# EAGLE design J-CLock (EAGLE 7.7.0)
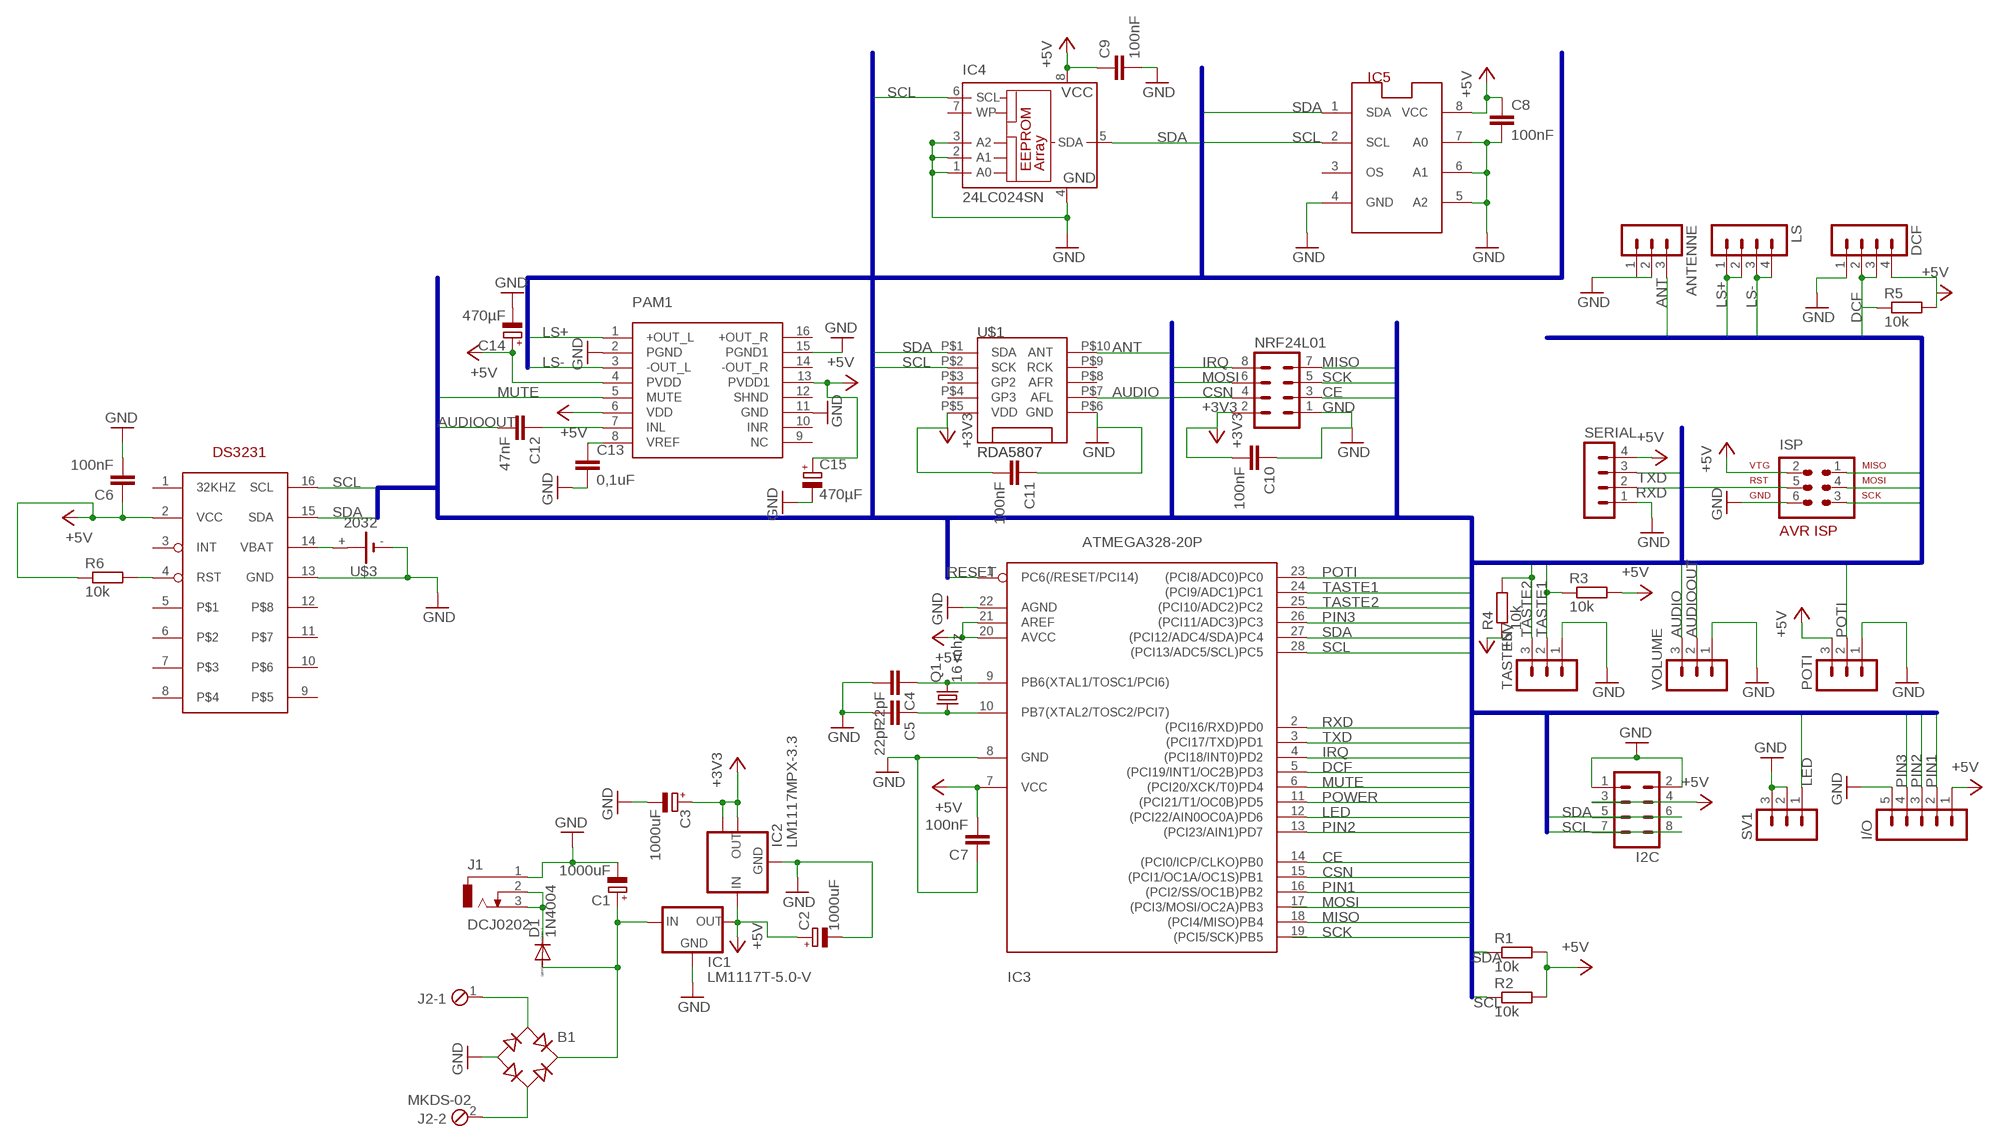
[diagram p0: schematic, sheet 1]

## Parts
ANTENNE  MA03-1  [MA03-1]
B1  B-DIL  [B-DIL]
C1  1000uF  CPOL-EUE5-10.5  [E5-10,5]
C2  1000uF  CPOL-EUE5-10.5  [E5-10,5]
C3  1000uF  CPOL-EUE5-10.5  [E5-10,5]
C4  22pF  C-EU050-030X075  [C050-030X075]
C5  22pF  C-EU050-030X075  [C050-030X075]
C6  100nF  C-EU050-030X075  [C050-030X075]
C7  100nF  C-EU050-030X075  [C050-030X075]
C8  100nF  C-EU050-030X075  [C050-030X075]
C9  100nF  C-EU050-030X075  [C050-030X075]
C10  100nF  C-EU050-030X075  [C050-030X075]
C11  100nF  C-EU050-030X075  [C050-030X075]
C12  47nF  C-EU050-030X075  [C050-030X075]
C13  0,1uF  C-EU050-030X075  [C050-030X075]
C14  470µF  CPOL-EUE3.5-8  [E3,5-8]
C15  470µF  CPOL-EUE3.5-8  [E3,5-8]
D1  1N4004  [DO41-10]
DCF  MA04-1  [MA04-1]
I2C  MA04-2  [MA04-2]
I/O  MA05-1  [MA05-1]
IC1  LM1117T-5.0-V  [TO220V]
IC2  LM1117MPX-3.3  [SOT223]
IC3  ATMEGA328-20P  [DIL28-3]
IC4  24LC024SN  [SO-08]
IC5  LM75_ICN  [SO8_LM75]
ISP  AVR-ISP-6  [AVR-ISP-6]
J1  DCJ0202  [DCJ0202]
J2  MKDS-02  [MKDS-02]
LS  MA04-1  [MA04-1]
NRF24L01  MA04-2  [MA04-2]
PAM1  PAM8403  [SOP-16]
POTI  MA03-1  [MA03-1]
Q1  16 mhz  CRYSTALHC49S  [HC49/S]
R1  10k  R-EU_0207/5V  [0207/5V]
R2  10k  R-EU_0207/5V  [0207/5V]
R3  10k  R-EU_0207/5V  [0207/5V]
R4  10k  R-EU_0207/5V  [0207/5V]
R5  10k  R-EU_0207/5V  [0207/5V]
R6  10k  R-EU_0207/5V  [0207/5V]
SERIAL  MA04-1  [MA04-1]
SV1  MA03-1  [MA03-1]
TASTEN  MA03-1  [MA03-1]
U$1  RDA5807  [RDA]
U$2  DS3231  [SO16]
U$3  2032  [KZH20SMD]
VOLUME  MA03-1  [MA03-1]

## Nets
+3V3: C3.+ C10.2 C11.2 IC2.2(OUT) IC2.TAB(OUT1) NRF24L01.2 U$1.P$5(VDD)
+5V: C2.+ C6.1 C7.2 C8.1 C9.1 C14.+ C15.+ DCF.4 I2C.3 I2C.4 I/O.1 IC1.2(OUT) IC2.3(IN) IC3.7(VCC) IC3.20(AVCC) IC3.21(AREF) IC4.8(VCC) IC5.8(VCC) ISP.2 PAM1.4(PVDD) PAM1.6(VDD) PAM1.13(PVDD1) POTI.3 R1.2 R2.2 R3.2 R4.1 R5.2 R6.1 SERIAL.4 U$2.2(VCC)
ANT: ANTENNE.3 U$1.P$10(ANT)
AUDIO: U$1.P$7(AFL) VOLUME.3
AUDIOOUT: C12.2 VOLUME.2
CE: IC3.14((PCI0/ICP/CLKO)PB0) NRF24L01.3
CSN: IC3.15((PCI1/OC1A/OC1S)PB1) NRF24L01.4
DCF: DCF.2 DCF.3 IC3.5((PCI19/INT1/OC2B)PD3) R5.1
GND: ANTENNE.1 ANTENNE.2 B1.- C1.- C2.- C3.- C4.2 C5.2 C6.2 C7.1 C8.2 C9.2 C10.1 C11.1 C13.2 C14.- C15.- DCF.1 I2C.1 I2C.2 I/O.5 IC1.1(GND) IC2.1(GND) IC3.8(GND) IC3.22(AGND) IC4.1(A0) IC4.2(A1) IC4.3(A2) IC4.4(GND) IC5.4(GND) IC5.5(A2) IC5.6(A1) IC5.7(A0) ISP.6 J1.1 NRF24L01.1 PAM1.2(PGND) PAM1.11(GND) PAM1.15(PGND1) POTI.1 SERIAL.1 SV1.2 SV1.3 TASTEN.1 U$1.P$6(GND) U$2.13(GND) U$3.- VOLUME.1
IRQ: IC3.4((PCI18/INT0)PD2) NRF24L01.8
LED: IC3.12((PCI22/AIN0OC0A)PD6) SV1.1
LS+: LS.1 LS.2 PAM1.1(+OUT_L)
LS-: LS.3 LS.4 PAM1.3(-OUT_L)
MISO: IC3.18((PCI4/MISO)PB4) ISP.1 NRF24L01.7
MOSI: ISP.4 NRF24L01.6
MUTE: IC3.6((PCI20/XCK/T0)PD4) PAM1.5(MUTE)
N$1: B1.AC2 J2.2
N$2: C4.1 IC3.9(PB6(XTAL1/TOSC1/PCI6)) Q1.2
N$3: B1.+ C1.+ D1.A IC1.3(IN)
N$4: C5.1 IC3.10(PB7(XTAL2/TOSC2/PCI7)) Q1.1
N$5: U$2.14(VBAT) U$3.+
N$6: D1.C J1.2 J1.3
N$7: B1.AC1 J2.1
N$8: R6.2 U$2.4(RST)
N$9: C12.1 PAM1.7(INL)
N$10: C13.1 PAM1.8(VREF)
PIN1: I/O.2 IC3.16((PCI2/SS/OC1B)PB2)
PIN2: I/O.3 IC3.13((PCI23/AIN1)PD7)
PIN3: I/O.4 IC3.26((PCI11/ADC3)PC3)
POTI: IC3.23((PCI8/ADC0)PC0) POTI.2
POWER: IC3.11((PCI21/T1/OC0B)PD5)
RESET: IC3.1(PC6(/RESET/PCI14)) ISP.5
RXD: IC3.2((PCI16/RXD)PD0) SERIAL.2
SCK: ISP.3 NRF24L01.5
SCL: I2C.7 I2C.8 IC3.28((PCI13/ADC5/SCL)PC5) IC4.6(SCL) IC5.2(SCL) R2.1 U$1.P$2(SCK) U$2.16(SCL)
SDA: I2C.5 I2C.6 IC3.27((PCI12/ADC4/SDA)PC4) IC4.5(SDA) IC5.1(SDA) R1.1 U$1.P$1(SDA) U$2.15(SDA)
TASTE1: IC3.24((PCI9/ADC1)PC1) R3.1 TASTEN.2
TASTE2: IC3.25((PCI10/ADC2)PC2) R4.2 TASTEN.3
TXD: IC3.3((PCI17/TXD)PD1) SERIAL.3
Unconnected: IC3.17((PCI3/MOSI/OC2A)PB3) IC3.19((PCI5/SCK)PB5) IC4.7(WP) IC5.3(OS) PAM1.9(NC) PAM1.10(INR) PAM1.12(SHND) PAM1.14(-OUT_R) PAM1.16(+OUT_R) U$1.P$3(GP2) U$1.P$4(GP3) U$1.P$8(AFR) U$1.P$9(RCK) U$2.1(32KHZ) U$2.3(INT) U$2.5 U$2.6 U$2.7 U$2.8 U$2.9 U$2.10 U$2.11 U$2.12

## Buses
CE,CSN,SCK,MOSI,MISO,IRQ,RESET,SDA,SCL,TXD,RXD,TASTE1,TASTE2,POTI,DCF,MUTE,POWER,LED,AUDIO,AUDIOOUT,LS+,LS-,ANT,PIN1,PIN2,PIN3

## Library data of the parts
ANTENNE POTI SV1 TASTEN VOLUME = con-lstb:MA03-1: PIN HEADER; OC_FARNELL: unknown; OC_NEWARK: unknown
B1 = rectifier:B-DIL: RECTIFIER
C1-C3 C14 C15 = resistor:CPOL-EU: POLARIZED CAPACITOR, European symbol
C4-C13 = resistor:C-EU: CAPACITOR, European symbol
D1 = diode:1N4004: DIODE
DCF LS SERIAL = con-lstb:MA04-1: PIN HEADER; OC_FARNELL: unknown; OC_NEWARK: unknown
I2C NRF24L01 = con-lstb:MA04-2: PIN HEADER; OC_FARNELL: unknown; OC_NEWARK: unknown
I/O = con-lstb:MA05-1: PIN HEADER; OC_FARNELL: unknown; OC_NEWARK: unknown
IC1 = lm1117:LM1117T-*
IC2 = lm1117:LM1117MPX-*
IC3 = atmega328:ATMEGA328*P: MICROCONTROLLER 32 kBytes FLASH 2 kBytes SRAM 1 kBytes EEPROM USART 8-channel 10 bit ADC
IC4 = microchip:24*: Serial EEPROM I2C; MF: MICROCHIP; MPN: 24LC024/SN; OC_FARNELL: 1659744; OC_NEWARK: 92C7092
IC5 = lm75:LM75_IC: Temperatursensor
ISP = avr-6:AVR-ISP-6: AVR ISP-6 Serial Programming Header
J1 = con-jack:DCJ0202: DC POWER JACK Source: DCJ0202.pdf; OC_FARNELL: unknown; OC_NEWARK: unknown
J2 = con-phoenix-500:MKDS-02: MKDSN COMBICON SERIES
PAM1 = PAM8403:PAM8403: Dual channel audio amplifier IC - PAM8403
Q1 = crystal:CRYSTAL: CRYSTAL; OC_FARNELL: 1667008; OC_NEWARK: unknown
R1-R6 = resistor:R-EU_: RESISTOR, European symbol
U$1 = RDA5807:RDA5807
U$2 = DS3231:DS3231
U$3 = kzh20_lithium_batterie_holder:2032

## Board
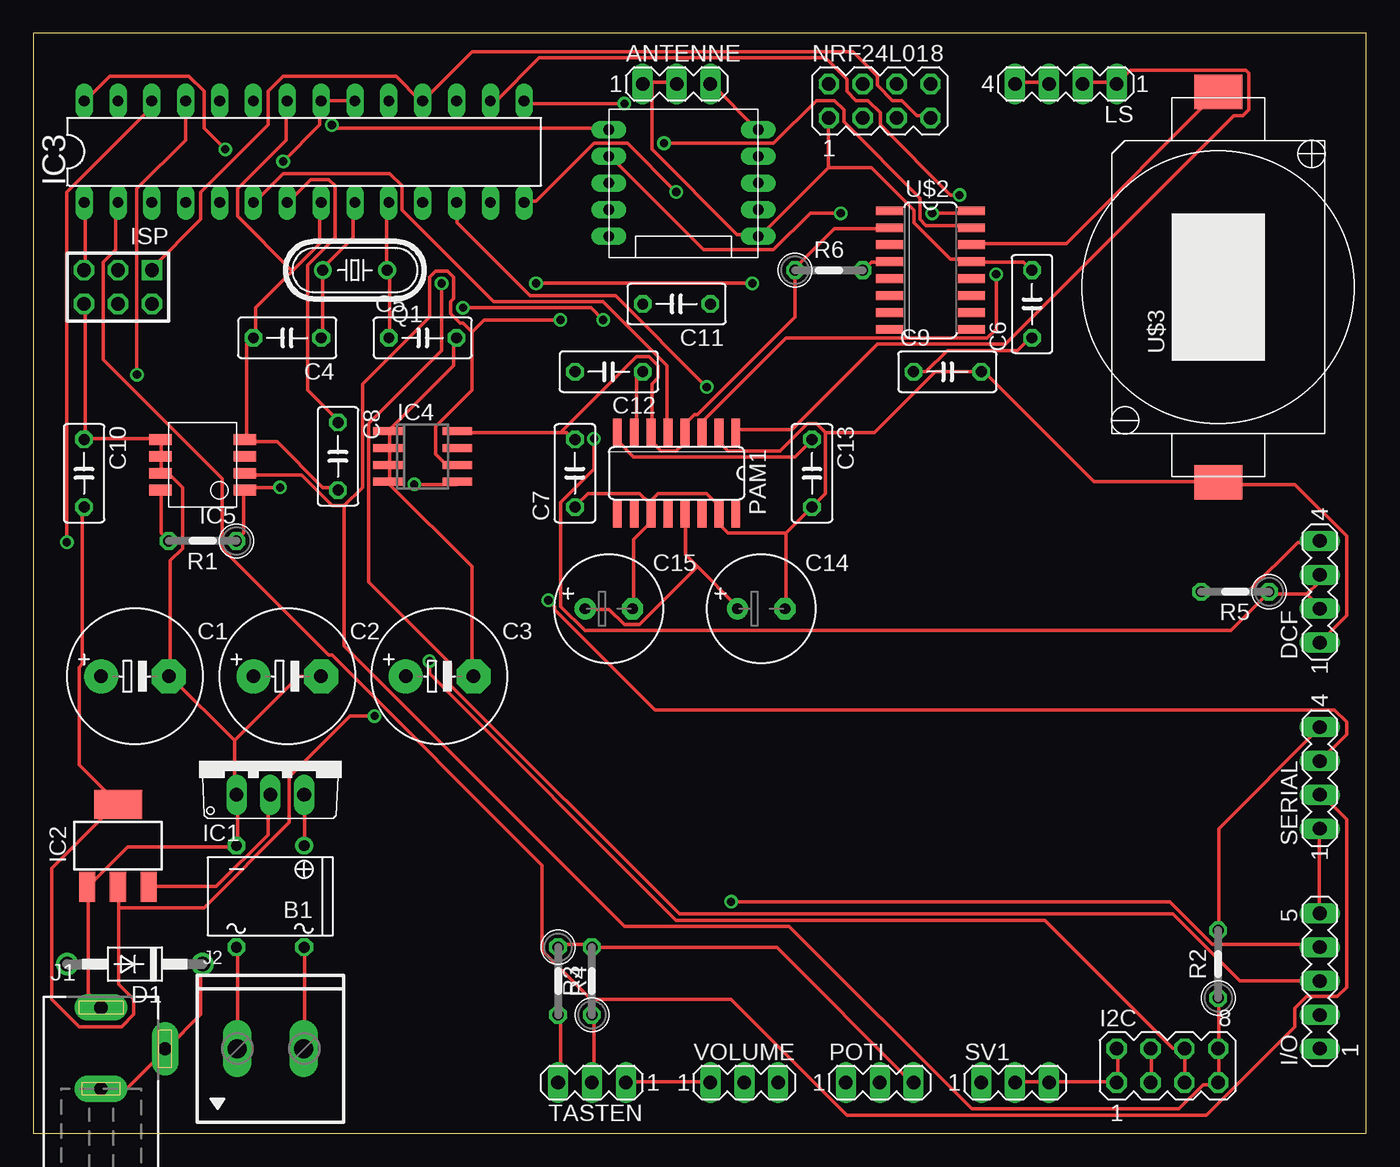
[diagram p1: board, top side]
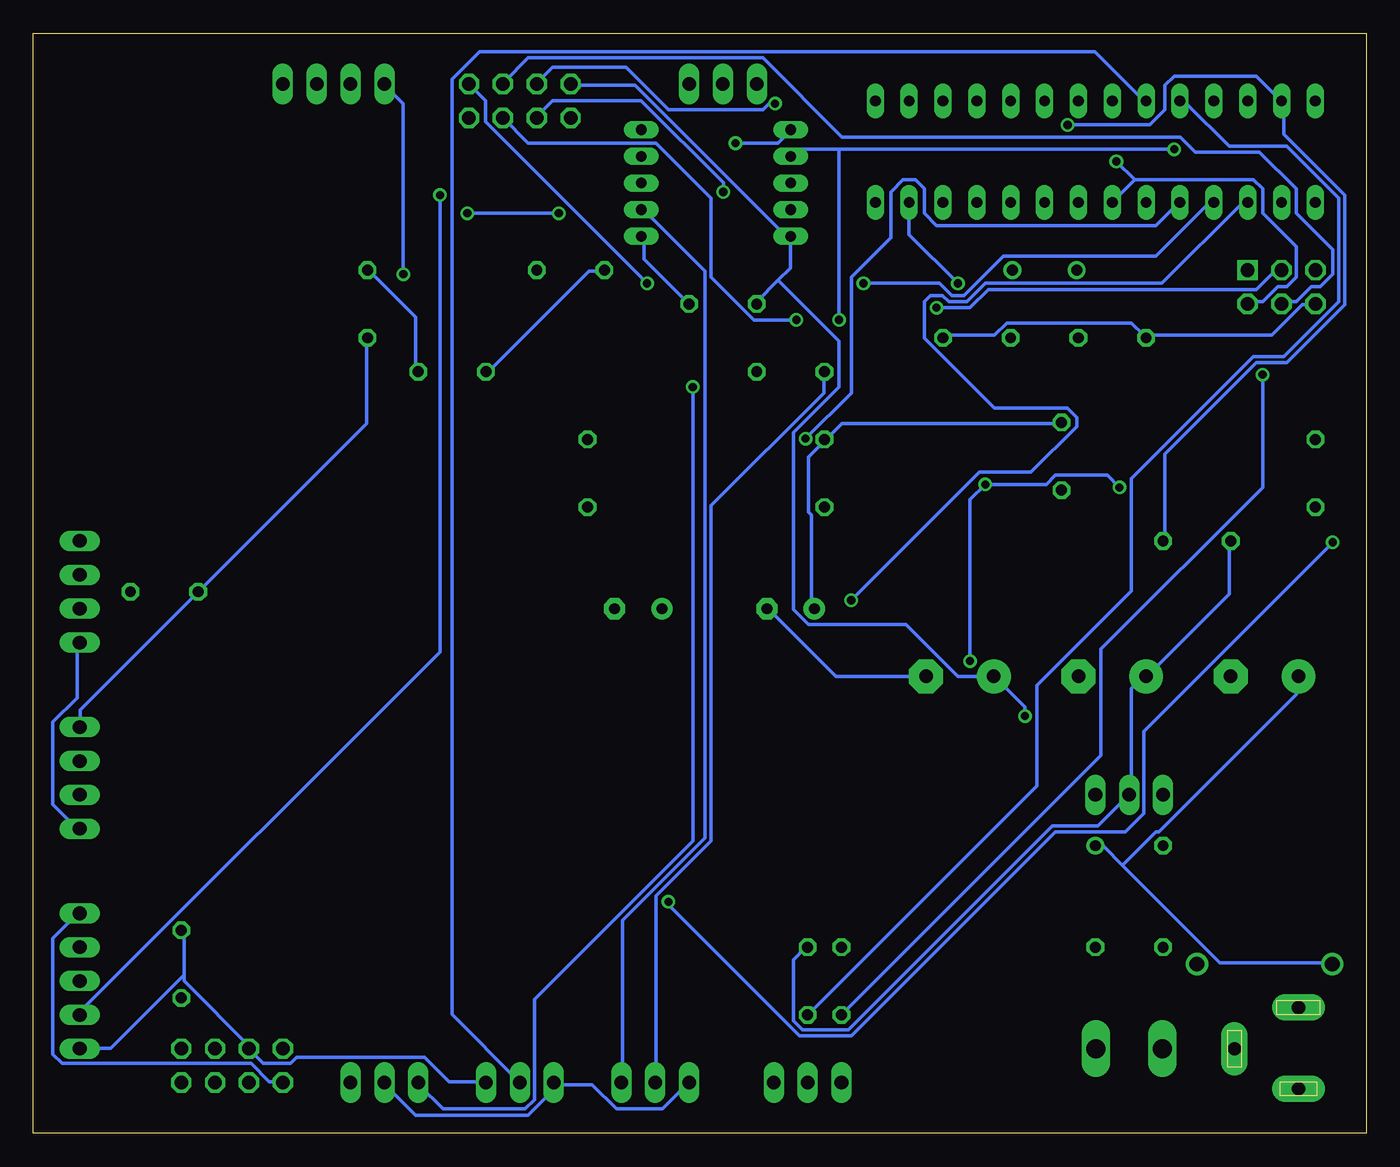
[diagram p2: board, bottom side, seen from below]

Size 100 x 82.54 mm. Coordinates in mm from the lower left corner, seen from the top.
Outline: 0,0 100,0 100,82.54 0,82.54 0,0
Copper layers (1*16): Top 0.035mm / dielectric 1.5mm / Bottom 0.035mm
Design rules "default": minimum track width 10mil, minimum drill 24mil, track to track 8mil, track to pad 8mil, pad to pad 8mil, via to via 8mil, smd to smd 8mil, copper to edge 40mil, drill to drill 8mil, minimum pad ring 10mil, minimum via ring 8mil, stop-mask expansion 4mil, vias tented up to drill 0mil, thermal gap 10mil

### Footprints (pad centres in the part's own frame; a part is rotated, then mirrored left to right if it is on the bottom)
MA03-1 = drill 1.016 long: 1 -2.54,0; 2 0,0; 3 2.54,0
B-DIL = drill 0.813: + -2.54,-3.81 | drill 0.813 octagon: - 2.54,-3.81; AC1 2.54,3.81; AC2 -2.54,3.81
E5-10,5 = drill 1.016 pad 2.54: + -2.54,0 | drill 1.016 pad 2.54 octagon: - 2.54,0
C050-030X075 = drill 0.813 octagon: 1 -2.54,0; 2 2.54,0
E3,5-8 = drill 0.813 pad 1.6: + -1.778,0 | drill 0.813 pad 1.6 octagon: - 1.778,0
DO41-10 = drill 1.118: A 5.08,0; C -5.08,0
MA04-1 = drill 1.016 long: 1 -3.81,0; 2 -1.27,0; 3 1.27,0; 4 3.81,0
MA04-2 = drill 1.016 octagon: 1 -3.81,-1.27; 2 -3.81,1.27; 3 -1.27,-1.27; 4 -1.27,1.27; 5 1.27,-1.27; 6 1.27,1.27; 7 3.81,-1.27; 8 3.81,1.27
MA05-1 = drill 1.016 long: 1 -5.08,0; 2 -2.54,0; 3 0,0; 4 2.54,0; 5 5.08,0
TO220V = drill 1.016 long: 1 -2.54,-2.54; 2 0,-2.54; 3 2.54,-2.54
SOT223 = smd 1.219 x 2.235: 1 -2.311,-3.099; 2 0,-3.099; 3 2.311,-3.099 | smd 3.6 x 2.2: TAB 0,3.099
DIL28-3 = drill 0.813 long: 1 -16.51,-3.81; 2 -13.97,-3.81; 3 -11.43,-3.81; 4 -8.89,-3.81; 5 -6.35,-3.81; 6 -3.81,-3.81; 7 -1.27,-3.81; 8 1.27,-3.81; 9 3.81,-3.81; 10 6.35,-3.81; 11 8.89,-3.81; 12 11.43,-3.81; 13 13.97,-3.81; 14 16.51,-3.81; 15 16.51,3.81; 16 13.97,3.81; 17 11.43,3.81; 18 8.89,3.81; 19 6.35,3.81; 20 3.81,3.81; 21 1.27,3.81; 22 -1.27,3.81; 23 -3.81,3.81; 24 -6.35,3.81; 25 -8.89,3.81; 26 -11.43,3.81; 27 -13.97,3.81; 28 -16.51,3.81
SO-08 = smd 0.6 x 2.2: 1 -1.905,-2.6; 2 -0.635,-2.6; 3 0.635,-2.6; 4 1.905,-2.6; 5 1.905,2.6; 6 0.635,2.6; 7 -0.635,2.6; 8 -1.905,2.6
SO8_LM75 = smd 0.813 x 1.676: 1 -1.27,-3.175; 2 0,-3.175; 3 1.27,-3.175; 4 2.54,-3.175; 5 2.54,3.175; 6 1.27,3.175; 7 0,3.175; 8 -1.27,3.175
AVR-ISP-6 = drill 1.016 square: 1 -2.54,-1.27 | drill 1.016 octagon: 2 -2.54,1.27; 3 0,-1.27; 4 0,1.27; 5 2.54,-1.27; 6 2.54,1.27
DCJ0202 = drill 1 pad 2 long: 1 0,3.1; 2 4.8,0; 3 0,-3
MKDS-02 = drill 1.422 long: 1 -2.5,0; 2 2.5,0
SOP-16 = smd 0.66 x 2.032: 1 -4.445,-3.073; 2 -3.175,-3.073; 3 -1.905,-3.073; 4 -0.635,-3.073; 5 0.635,-3.073; 6 1.905,-3.073; 7 3.175,-3.073; 8 4.445,-3.073; 9 4.445,3.073; 10 3.175,3.073; 11 1.905,3.073; 12 0.635,3.073; 13 -0.635,3.073; 14 -1.905,3.073; 15 -3.175,3.073; 16 -4.445,3.073
HC49/S = drill 0.813: 1 -2.413,0; 2 2.413,0
0207/5V = drill 0.813 octagon: 1 -2.54,0; 2 2.54,0
RDA = drill 0.8 pad 1.265 long: P$1 0,8; P$2 0,6; P$3 0,4; P$4 0,2; P$5 0,0; P$6 11.2,0; P$7 11.2,2; P$8 11.2,4; P$9 11.2,6; P$10 11.2,8
SO16 = smd 0.66 x 2.032: 1 -4.445,-3.073; 2 -3.175,-3.073; 3 -1.905,-3.073; 4 -0.635,-3.073; 5 0.635,-3.073; 6 1.905,-3.073; 7 3.175,-3.073; 8 4.445,-3.073; 9 4.445,3.073; 10 3.175,3.073; 11 1.905,3.073; 12 0.635,3.073; 13 -0.635,3.073; 14 -1.905,3.073; 15 -3.175,3.073; 16 -4.445,3.073
KZH20SMD = smd 2.6 x 3.6: + 14.65,0; - -14.65,0

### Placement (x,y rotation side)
ANTENNE  48.26,78.74 0 top
B1  17.78,17.78 180 top
C1  7.62,34.29 0 top
C2  19.05,34.29 0 top
C3  30.48,34.29 0 top
C4  19.05,59.69 180 top
C5  29.21,59.69 0 top
C6  74.93,62.23 90 top
C7  40.64,49.53 90 top
C8  22.86,50.8 270 top
C9  68.58,57.15 0 top
C10  3.81,49.53 270 top
C11  48.26,62.23 180 top
C12  43.18,57.15 180 top
C13  58.42,49.53 270 top
C14  54.61,39.37 0 top
C15  43.18,39.37 0 top
D1  7.62,12.7 180 top
DCF  96.52,40.64 90 top
I2C  85.09,5.08 0 top
I/O  96.52,11.43 90 top
IC1  17.78,27.94 0 top
IC2  6.35,21.59 0 top
IC3  20.32,73.66 0 top
IC4  29.21,50.8 270 top
IC5  12.7,49.53 90 top
ISP  6.35,63.5 180 top
J1  5.08,6.35 0 top
J2  17.78,6.35 0 top
LS  77.47,78.74 180 top
NRF24L01  63.5,77.47 0 top
PAM1  48.26,49.53 180 top
POTI  63.5,3.81 0 top
Q1  24.13,64.77 180 top
R1  12.7,44.45 180 top
R2  88.9,12.7 90 top
R3  41.91,11.43 90 top
R4  39.37,11.43 270 top
R5  90.17,40.64 180 top
R6  59.69,64.77 0 top
SERIAL  96.52,26.67 90 top
SV1  73.66,3.81 0 top
TASTEN  41.91,3.81 180 top
U$1  43.18,67.31 0 top
U$2  67.31,64.77 270 top
U$3  88.9,63.5 90 top
VOLUME  53.34,3.81 0 top

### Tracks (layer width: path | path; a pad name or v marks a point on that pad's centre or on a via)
+3V3  (via drill 0.61)
  Top 0.254: 6.4,16.92 6.4,11.2 7.54,10.06 7.54,8.91 6.63,8 3.43,8 1.37,10.06 1.37,19.89 6.17,24.69 IC2.TAB 6.17,24.92 3.43,27.66 3.43,34.98 3.66,35.2 3.66,46.86 C10.2 | 6.4,16.92 6.4,18.29 IC2.2 | 6.4,16.92 12.8,16.92 19.2,23.32 19.2,26.75 23.77,31.32 v25.6,31.32
  Bottom 0.254: 43.2,66.98 43.2,64.92 44.12,64.01 | 43.2,66.98 43.2,67.21 U$1.P$5 43.2,66.98 | 44.12,64.01 45.72,62.41 C11.2 | 43.2,66.98 54.86,78.64 59.66,78.64 NRF24L01.2 | 44.12,64.01 39.55,59.44 39.55,56.01 42.98,52.58 42.98,39.32 41.83,38.18 34.52,38.18 30.63,34.29 C3.+ 27.89,34.29 25.6,32 v25.6,31.32
+5V  (via drill 0.61)
  Top 0.254: U$2.2 64.24,67.89 60.12,67.89 57.15,64.92 R6.1 57.15,61.27 49.84,53.95 49.61,53.95 48.92,53.26 48.92,52.81 PAM1.4 48.69,52.58 48.69,51.66 48.23,51.21 47.09,51.21 46.41,51.89 46.41,52.58 PAM1.6 46.41,52.81 46.41,56.24 46.86,56.69 46.86,57.61 46.18,58.29 45.26,58.29 39.55,52.58 | C9.1 66.98,57.15 68.58,58.75 73.84,58.75 74.75,59.66 C6.1 | 49.84,42.52 52.81,39.55 C14.+ | 49.84,42.52 48.92,43.43 48.92,46.41 PAM1.13 | 49.84,42.52 45.49,38.18 44.35,38.18 43.2,39.32 41.6,39.32 C15.+ | IC3.20 24,77.5 21.72,77.5 IC3.21 21.49,77.27 21.49,75.67 v18.75,72.92 | 39.55,52.58 40.01,52.58 40.46,52.12 C7.2 | 39.55,52.58 32,52.58 IC4.8 | IC3.7 19.2,69.95 20.8,71.55 22.17,71.55 22.63,71.09 22.63,67.21 20.57,65.15 20.57,55.78 22.86,53.49 C8.1 | IC2.3 8.69,18.52 13.72,18.52 17.6,22.4 17.6,25.38 IC1.2 | IC5.8 9.6,48.23 9.6,45.03 10.06,44.58 R1.2 | R5.2 87.78,40.69 91.21,40.69 94.87,44.35 96.47,44.35 DCF.4 | R4.1 39.55,14.17 41.83,14.17 R3.2 42.06,13.95 55.78,13.95 65.84,3.89 POTI.3 | I2C.3 83.9,3.89 83.9,6.17 I2C.4 | SERIAL.4 96.47,30.4 88.92,22.86 88.92,15.32 R2.2
  Bottom 0.254: R6.1 57.15,64.69 58.29,64.69 65.84,57.15 C9.1 | C8.1 22.86,53.26 39.32,53.26 40.46,52.12 C7.2 40.69,51.89 41.83,50.75 41.83,46.63 41.6,46.41 41.6,39.55 C15.+ | 17.37,71.55 8.46,71.55 7.77,70.87 7.77,69.04 5.26,66.52 5.26,64.24 5.94,63.55 6.63,63.55 7.77,62.41 8.69,62.41 ISP.2 | 17.37,71.55 18.97,69.95 IC3.7 | 17.37,71.55 v18.75,72.92 | R1.2 10.29,44.35 10.29,40.46 16.46,34.29 C2.+ 16.69,34.29 17.6,33.38 17.6,25.6 IC1.2 17.83,25.38 20.12,23.09 23.55,23.09 38.86,7.77 42.29,7.77 42.98,8.46 42.98,13.03 42.06,13.95 R3.2 | SERIAL.4 96.47,30.63 96.47,31.77 87.78,40.46 R5.2 87.55,40.69 74.98,53.26 74.98,59.66 C6.1 | 88.7,11.89 88.7,11.43 83.67,6.4 I2C.4 83.67,6.17 82.75,5.26 80.7,5.26 80.24,5.71 70.64,5.71 68.81,3.89 66.06,3.89 POTI.3 | 88.7,11.89 88.7,15.09 R2.2 | 88.7,11.89 94.18,6.4 96.47,6.4 I/O.1
ANT
  Top 0.254: U$1.P$10 54.18,75.44 50.98,78.64 ANTENNE.3
AUDIO
  Bottom 0.254: U$1.P$7 54.18,69.27 49.61,64.69 49.61,22.17 55.78,16 55.78,3.89 VOLUME.3
AUDIOOUT
  Bottom 0.254: C12.2 40.69,57.15 40.69,55.55 49.15,47.09 49.15,21.95 53.26,17.83 53.26,3.89 VOLUME.2
CE  (via drill 0.61)
  Top 0.254: v48.23,70.64 44.58,74.3 42.06,74.3 37.72,69.95 37.03,69.95 IC3.14
  Bottom 0.254: v48.23,70.64 48.23,71.32 54.41,77.5 61.04,77.5 62.18,76.35 NRF24L01.3
CSN  (via drill 0.61)
  Top 0.254: v44.35,77.27 37.03,77.27 IC3.15
  Bottom 0.254: v44.35,77.27 44.81,77.27 45.26,76.81 52.35,76.81 55.55,80.01 61.04,80.01 62.18,78.87 NRF24L01.4
DCF  (via drill 0.61)
  Top 0.254: 95.56,40.46 92.81,40.46 R5.1 92.58,40.46 89.84,37.72 41.38,37.72 39.55,39.55 39.55,47.32 42.06,49.84 v42.06,52.12 | 95.56,40.46 96.47,39.55 DCF.2 | 95.56,40.46 96.47,41.38 96.47,41.83 DCF.3
  Bottom 0.254: v42.06,52.12 38.63,55.55 38.63,64.24 35.66,67.21 35.66,70.64 34.75,71.55 33.83,71.55 33.15,70.87 33.15,69.04 32.23,68.12 15.77,68.12 14.17,69.72 IC3.5
GND
  Top 0.254: SV1.2 73.84,3.89 76.12,3.89 SV1.3 76.35,3.89 81.15,3.89 I2C.1 81.38,3.89 81.38,6.17 I2C.2 | TASTEN.1 44.58,3.89 50.75,3.89 VOLUME.1 | I/O.5 96.47,16.69 96.47,22.86 SERIAL.1 | DCF.1 96.7,37.03 98.53,38.86 98.53,44.81 94.64,48.69 88.92,48.69 U$3.- 88.7,48.92 79.55,48.92 71.32,57.15 C9.2 67.67,57.15 63.09,52.58 59.44,52.58 | 46.18,47.32 46.18,46.63 PAM1.11 | 46.18,47.32 45.49,48.01 41.6,48.01 40.69,47.09 C7.1 | 46.18,47.32 46.86,48.01 50.52,48.01 51.44,47.09 PAM1.15 51.44,45.72 52.12,45.03 56.46,45.03 | 46.18,47.32 PAM1.11 | C15.- 45.03,39.55 45.03,44.58 46.18,45.72 46.18,46.41 PAM1.11 | 46.41,78.87 48.23,78.87 ANTENNE.2 | 46.41,78.87 45.72,78.87 ANTENNE.1 46.41,78.87 | 59.66,72.47 59.66,76.12 NRF24L01.1 | 59.66,72.47 54.41,67.21 U$1.P$6 54.18,67.44 52.81,67.44 46.41,73.84 46.41,78.87 | C6.2 74.75,64.92 74.3,65.38 70.41,65.38 U$2.13 70.18,65.61 68.81,65.61 66.06,68.35 66.06,69.27 62.87,72.47 59.66,72.47 | PAM1.2 51.44,51.89 52.12,51.21 56.01,51.21 58.06,53.26 58.75,53.26 59.44,52.58 | 59.44,52.58 59.44,48.01 C13.2 56.46,45.03 | 56.46,45.03 56.46,39.55 C14.- | J1.1 5.03,9.6 4.12,10.52 4.12,18.29 IC2.1 4.12,18.52 7.09,21.49 15.09,21.49 B1.- 15.32,21.72 15.32,25.38 IC1.1 15.09,25.6 15.09,29.49 | 10.29,34.29 15.09,29.49 | C2.- 19.89,34.29 15.09,29.49 | 3.89,52.12 9.37,52.12 IC5.5 9.6,51.89 9.6,50.98 IC5.6 9.6,50.75 9.6,49.61 IC5.7 9.6,49.38 10.29,49.38 11.2,48.46 11.2,43.89 10.29,42.98 10.29,34.29 | 3.89,52.12 3.89,62.18 ISP.6 | 3.89,52.12 C10.1 | 26.75,51.44 26.75,52.58 IC4.1 26.75,52.81 31.55,57.61 31.55,59.66 C5.2 | 26.75,51.44 26.75,50.29 IC4.3 26.75,50.06 26.75,48.92 IC4.4 26.75,48.69 32.92,42.52 32.92,34.29 C3.-
  Top 0.254: 26.75,51.44 IC4.2 | C8.2 22.86,48.46 21.72,48.46 18.29,51.89 16,51.89 IC5.4 16,52.12 16,59.21 16.46,59.66 C4.2 16.69,59.89 16.69,61.95 19.43,64.69 | 19.43,64.69 21.49,66.75 21.49,69.72 IC3.8 | 19.43,64.69 15.32,68.81 15.32,70.87 18.97,74.52 18.97,77.27 IC3.22 | 10.29,34.29 C1.-
  Bottom 0.254: 60.58,3.66 58.06,3.66 56.24,1.83 52.81,1.83 50.98,3.66 VOLUME.1 | 60.58,3.66 60.81,3.66 POTI.1 60.58,3.66 | 60.58,3.66 62.87,1.37 71.32,1.37 73.61,3.66 SV1.2 | DCF.1 96.7,36.8 96.7,32.69 98.53,30.86 98.53,24.69 96.7,22.86 SERIAL.1 | I2C.1 81.38,3.89 82.3,3.89 83.67,5.26 97.84,5.26 98.53,5.94 98.53,14.63 96.7,16.46 I/O.5 | C3.- 39.78,34.29 44.81,39.32 C15.- | C11.1 54.18,65.61 54.18,67.21 U$1.P$6 | C9.2 71.32,57.15 71.32,61.27 74.75,64.69 C6.2 | C5.2 31.55,59.89 27.89,59.89 26.98,60.81 17.6,60.81 16.69,59.89 C4.2 16.46,59.89 7.09,59.89 4.8,62.18 3.89,62.18 ISP.6
IRQ  (via drill 0.61)
  Top 0.254: v53.95,63.78 v37.72,63.78
  Bottom 0.254: v37.72,63.78 32,63.78 31.09,62.87 30.18,62.87 27.2,65.84 15.77,65.84 11.89,69.72 11.43,69.72 IC3.4 | v53.95,63.78 66.06,75.89 66.06,77.5 NRF24L01.8
LED  (via drill 0.61)
  Top 0.254: v50.52,56.01 43.66,62.87 37.26,62.87 31.77,68.35 31.77,69.72 IC3.12
  Bottom 0.254: v50.52,56.01 50.52,21.95 62.41,10.06 62.41,2.52 63.09,1.83 69.27,1.83 71.09,3.66 SV1.1
LS+
  Top 0.254: PAM1.1 52.81,52.81 56.92,52.81 63.32,59.21 72.92,59.21 90.07,76.35 90.75,76.35 91.21,76.81 91.21,79.55 90.98,79.78 82.3,79.78 81.38,78.87 LS.1 81.15,78.87 78.87,78.87 LS.2
LS-  (via drill 0.61)
  Top 0.254: v72.24,64.47 72.24,60.35 71.55,59.66 56.46,59.66 50.29,53.49 50.29,52.81 PAM1.3 | LS.3 76.12,78.87 73.84,78.87 LS.4
  Bottom 0.254: v72.24,64.47 72.24,77.27 73.61,78.64 LS.4
MISO
  Top 0.254: ISP.1 8.91,64.92 12.57,68.58 12.57,70.64 17.6,75.67 17.6,78.18 18.75,79.32 27.2,79.32 29.03,77.5 IC3.18 29.26,77.5 32.92,81.15 61.49,81.15 63.32,79.32 63.32,78.64 64.47,77.5 65.15,77.5 66.29,76.35 67.21,76.35 NRF24L01.7
MOSI
  Bottom 0.254: ISP.4 6.17,62.41 5.26,62.41 4.12,63.55 3.43,63.55 2.52,64.47 2.52,66.29 5.26,69.04 5.26,70.87 8,73.61 12.8,73.61 13.95,74.75 39.32,74.75 45.26,80.7 62.87,80.7 64.69,78.87 NRF24L01.6
MUTE
  Top 0.254: PAM1.5 47.55,52.81 47.55,57.61 42.75,62.41 34.52,62.41 27.66,69.27 27.66,71.09 26.75,72.01 18.75,72.01 16.69,69.95 IC3.6
N$1
  Top 0.254: B1.AC2 20.34,13.95 20.34,6.4 J2.2
N$2
  Top 0.254: C4.1 21.72,59.89 Q1.2 21.72,64.92 24,67.21 24,69.72 IC3.9
N$3
  Top 0.254: B1.+ 20.34,21.72 20.34,25.38 IC1.3
  Bottom 0.254: 18.29,20.12 19.66,21.49 20.12,21.49 B1.+ | 18.29,20.12 10.97,12.8 2.74,12.8 D1.A | 18.29,20.12 15.77,22.63 15.54,22.63 5.26,32.92 5.26,34.29 C1.+
N$4
  Top 0.254: IC3.10 26.52,69.72 26.52,64.92 Q1.1 26.75,64.69 26.75,59.89 C5.1
N$5
  Top 0.254: U$2.14 70.41,66.75 77.5,66.75 88.7,77.95 U$3.+
N$6
  Top 0.254: D1.C 12.57,12.57 12.57,8.91 10.06,6.4 J1.2 9.83,6.17 7.09,3.43 5.26,3.43 J1.3
N$7
  Top 0.254: B1.AC1 15.32,13.95 15.32,6.4 J2.1
N$8
  Top 0.254: U$2.4 64.24,65.38 62.87,65.38 62.41,64.92 R6.2
N$9
  Top 0.254: C12.1 45.26,56.69 45.26,52.81 PAM1.7
N$10
  Top 0.254: PAM1.8 43.89,52.58 43.89,51.89 45.03,50.75 57.15,50.75 58.29,51.89 C13.1
PIN1  (via drill 0.61)
  Top 0.254: v69.49,70.41 68.81,70.41 63.55,75.67 63.55,76.58 62.64,77.5 61.72,77.5 61.04,78.18 61.04,79.1 59.44,80.7 37.95,80.7 34.75,77.5 34.29,77.5 IC3.16
  Bottom 0.254: v69.49,70.41 69.49,36.12 96.7,8.91 I/O.2
PIN2  (via drill 0.61)
  Top 0.254: v30.63,63.78 30.63,58.75 25.15,53.26 25.15,41.38 31.32,35.2 31.32,33.6 48.46,16.46 85.5,16.46 90.53,11.43 I/O.3
  Bottom 0.254: IC3.13 34.29,67.44 v30.63,63.78
PIN3  (via drill 0.61)
  Top 0.254: v2.52,44.35 2.52,70.64 8.69,76.81 8.69,77.27 IC3.26 | v52.35,17.37 85.27,17.37 88.47,14.17 96.47,14.17 I/O.4
  Bottom 0.254: v2.52,44.35 16.69,30.18 16.69,24 18.06,22.63 23.32,22.63 38.63,7.32 42.52,7.32 52.35,17.14 v52.35,17.37
POTI
  Bottom 0.254: IC3.23 16.69,77.5 20.34,81.15 66.52,81.15 68.58,79.1 68.58,8.91 63.55,3.89 POTI.2
RESET
  Top 0.254: IC3.1 3.89,69.72 3.89,64.92 ISP.5
RXD
  Top 0.254: IC3.2 6.17,69.72 6.17,66.29 5.26,65.38 5.26,58.06 14.17,49.15 14.17,43.89 22.17,35.89 22.4,35.89 38.18,20.12 38.18,13.72 41.83,10.06 52.35,10.06 61.04,1.37 88.01,1.37 94.64,8 94.64,9.37 95.56,10.29 97.84,10.29 98.53,10.97 98.53,23.55 96.7,25.38 SERIAL.2
SCK  (via drill 0.61)
  Top 0.254: v32.23,61.95 41.83,61.95 v42.75,61.04
  Bottom 0.254: v32.23,61.95 29.72,61.95 28.35,63.32 8.23,63.32 6.86,64.69 6.4,64.69 ISP.3 | v42.75,61.04 45.95,61.04 49.15,64.24 49.15,70.18 53.26,74.3 62.87,74.3 NRF24L01.5
SCL  (via drill 0.61)
  Top 0.254: v67.44,69.04 70.18,69.04 U$2.16 | v60.58,69.04 58.29,69.04 55.55,66.29 50.29,66.29 43.2,73.38 U$1.P$2 | v14.4,73.84 12.8,75.44 12.8,78.18 11.66,79.32 5.71,79.32 3.89,77.5 IC3.28 | R2.1 88.92,10.06 88.92,6.4 I2C.8 88.92,6.17 88.92,3.89 I2C.7 88.7,3.66 87.78,3.66 85.95,1.83 70.41,1.83 56.69,15.54 44.35,15.54 23.32,36.58 23.32,47.09 | 23.32,47.09 22.4,47.09 20.12,49.38 16,49.38 IC5.2 | 23.32,47.09 24.69,48.46 24.69,56.24 29.72,61.27 29.72,64.24 30.18,64.69 31.09,64.69 31.55,64.24 31.55,62.64 31.32,62.41 31.32,61.49 32,60.81 32.23,60.81 32.92,60.12 | 32.92,60.12 32.92,55.78 30.18,53.03 30.18,50.98 30.86,50.29 31.77,50.29 IC4.6 | v39.55,61.04 33.83,61.04 32.92,60.12
  Bottom 0.254: v60.58,69.04 v67.44,69.04 | 39.55,73.84 42.52,73.84 42.98,73.38 U$1.P$2 | 39.55,73.84 v14.4,73.84 | v39.55,61.04 39.55,73.84
SDA  (via drill 0.61)
  Top 0.254: v47.32,74.3 55.55,74.3 58.75,77.5 60.12,77.5 60.81,76.81 60.81,75.89 66.52,70.18 66.52,68.58 66.98,68.12 70.18,68.12 U$2.15 | I2C.5 86.41,3.89 86.41,6.17 I2C.6 86.18,6.4 85.5,6.4 75.89,16 48.23,16 29.72,34.52 v29.72,35.43 | R1.1 15.32,44.58 15.77,45.03 15.77,48.23 IC5.1 16,48.46 v18.52,48.46 | v28.57,48.69 31.77,48.69 IC4.5 | v22.4,75.67 22.63,75.44 42.98,75.44 U$1.P$1
  Bottom 0.254: v47.32,74.3 44.12,74.3 43.2,75.21 U$1.P$1 | v18.52,48.46 19.43,49.38 23.32,49.38 24,48.69 v28.57,48.69 29.72,47.55 v29.72,35.43 | R1.1 15.09,44.58 15.09,50.98 8.23,57.84 5.94,57.84 1.6,62.18 1.6,70.41 6.17,74.98 6.17,77.27 IC3.27 6.4,77.5 8.23,79.32 14.4,79.32 15.09,78.64 15.09,76.81 16.23,75.67 v22.4,75.67
TASTE1
  Top 0.254: R3.1 42.06,8.69 42.06,3.89 TASTEN.2
  Bottom 0.254: IC3.24 13.95,77.27 13.49,77.27 10.29,74.07 5.94,74.07 2.06,70.18 2.06,62.41 6.17,58.29 8.46,58.29 17.6,49.15 17.6,40.69 24.69,33.6 24.69,26.06 41.83,8.91 R3.1
TASTE2  (via drill 0.61)
  Top 0.254: R4.2 39.55,8.69 39.55,3.89 TASTEN.3 | IC3.25 11.43,74.52 7.77,70.87 v7.77,56.92
  Bottom 0.254: v7.77,56.92 7.77,48.46 19.89,36.35 19.89,28.35 39.32,8.91 R4.2
TXD  (via drill 0.61)
  Top 0.254: v38.63,40.01 39.09,39.55 39.09,39.32 46.63,31.77 97.61,31.77 98.53,30.86 98.53,29.95 SERIAL.3
  Bottom 0.254: v38.63,40.01 29.03,49.61 25.15,49.61 21.72,53.03 21.72,53.72 22.4,54.41 27.89,54.41 33.15,59.66 33.15,62.41 32.69,62.87 31.77,62.87 31.32,62.41 29.95,62.41 28.57,63.78 15.32,63.78 9.37,69.72 8.91,69.72 IC3.3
